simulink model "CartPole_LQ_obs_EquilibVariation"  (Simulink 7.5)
settings: Solver=ode45  StartTime=0.0  StopTime=10.0  MaxStep=1e-2  RelTol=1e-3
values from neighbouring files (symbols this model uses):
  g = 9.81    [Exercises05.m]
  K = lqr(A,B,C'*Q*C,R)    [Exercises05.m]
  L = 1    [Exercises05.m]
  Lobs = - place(A',C',[-20 -20 -25 -25])'    [Exercises05.m]
  m = 0.1    [Exercises05.m]
  M = 1    [Exercises05.m]
  ue = 0    [Exercises05.m]
  X0 = Xe + dX0    [Exercises05.m]
undefined symbols (not defined in the file or in its folder): A, B, C

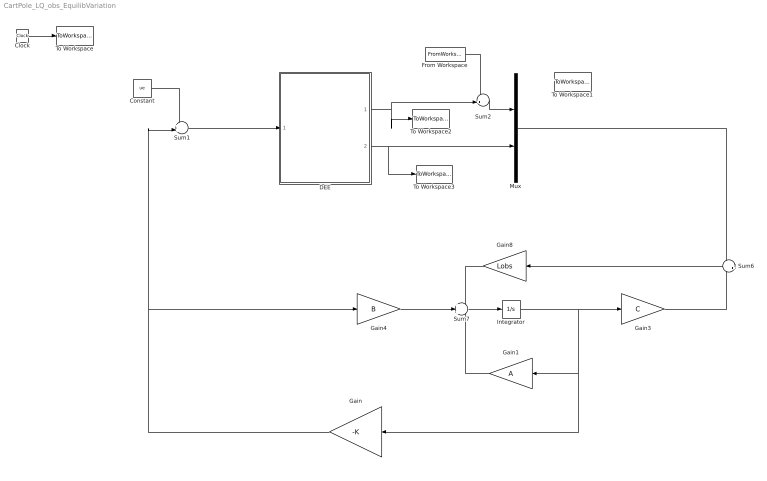
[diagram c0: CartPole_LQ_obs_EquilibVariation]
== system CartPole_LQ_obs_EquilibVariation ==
  Clock : Clock
  Constant : Constant  Value=ue  OutDataType=fixdt(1, 16)  OutScaling=2^0
  DEE : Subsystem
  From Workspace : FromWorkspace  VariableName=[t' Xe_t']  SampleTime=0
  Gain : Gain  Gain=-K  Multiplication=Matrix(K*u)  ParameterDataType=fixdt(1, 16)  ParameterScaling=2^0  OutDataType=fixdt(1, 16)  OutScaling=2^0
  Gain1 : Gain  Gain=A  Multiplication=Matrix(K*u)  ParameterDataType=sfix(16)  ParameterScaling=2^0  OutDataType=sfix(16)  OutScaling=2^0
  Gain3 : Gain  Gain=C  Multiplication=Matrix(K*u)  ParameterDataType=sfix(16)  ParameterScaling=2^0  OutDataType=sfix(16)  OutScaling=2^0
  Gain4 : Gain  Gain=B  Multiplication=Matrix(K*u)  ParameterDataType=sfix(16)  ParameterScaling=2^0  OutDataType=sfix(16)  OutScaling=2^0
  Gain8 : Gain  Gain=Lobs  Multiplication=Matrix(K*u)  ParameterDataType=sfix(16)  ParameterScaling=2^0  OutDataType=sfix(16)  OutScaling=2^0
  Integrator : Integrator  InitialCondition=[0 0 0 0]'
  Mux : Mux  Inputs=2
  Sum1 : Sum  Inputs=++|  OutDataType=fixdt(1, 16)  OutScaling=2^0
  Sum2 : Sum  Inputs=-+|  OutDataType=fixdt(1, 16)  OutScaling=2^0
  Sum6 : Sum  Inputs=-+  OutDataType=sfix(16)  OutScaling=2^0
  Sum7 : Sum  Inputs=+++  OutDataType=sfix(16)  OutScaling=2^0
  To Workspace : ToWorkspace  VariableName=time  SampleTime=-1  SaveFormat=Array
  To Workspace1 : ToWorkspace  VariableName=y  SampleTime=-1  SaveFormat=Array
  To Workspace2 : ToWorkspace  VariableName=y_1  SampleTime=-1  SaveFormat=Array
  To Workspace3 : ToWorkspace  VariableName=y_2  SampleTime=-1  SaveFormat=Array
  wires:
  Clock/1 -> To Workspace/1
  Gain/1 -> Sum1/2, Gain4/1
  Constant/1 -> Sum1/1
  Integrator/1 -> Gain3/1, Gain1/1, Gain/1
  Sum7/1 -> Integrator/1
  Gain3/1 -> Sum6/2
  Sum6/1 -> Gain8/1
  Gain8/1 -> Sum7/1
  Gain1/1 -> Sum7/3
  Gain4/1 -> Sum7/2
  Sum1/1 -> DEE/1(SysInport1)
  DEE/2(Port2) -> Mux/2, To Workspace3/1
  Mux/1 -> Sum6/1
  DEE/1(Port1) -> Sum2/2, To Workspace2/1
  Sum2/1 -> Mux/1
  From Workspace/1 -> Sum2/1

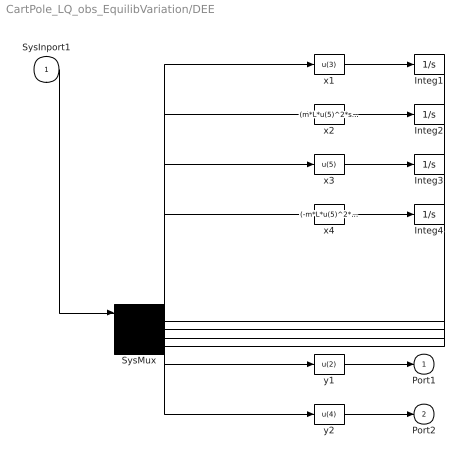
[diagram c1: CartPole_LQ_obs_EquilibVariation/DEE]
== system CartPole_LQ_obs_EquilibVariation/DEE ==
  SysInport1 : Inport
  Integ1 : Integrator  InitialCondition=X0(1)
  Integ2 : Integrator  InitialCondition=X0(2)
  Integ3 : Integrator  InitialCondition=X0(3)
  Integ4 : Integrator  InitialCondition=X0(4)
  SysMux : Mux  Inputs=5
  x1 : Fcn  Expr=u(3)
  x2 : Fcn  Expr=(m*L*u(5)^2*sin(u(4)) - m*g*sin(u(4))*cos(u(4))+ u)/(M+m*sin(u(4))^2)
  x3 : Fcn  Expr=u(5)
  x4 : Fcn  Expr=(-m*L*u(5)^2*sin(u(4))*cos(u(4))+(M+m)*g*sin(u(4))-u*cos(u(4)))/((M+m*sin(u(4))^2)*L)
  y1 : Fcn  Expr=u(2)
  y2 : Fcn  Expr=u(4)
  Port1 : Outport
  Port2 : Outport  Port=2
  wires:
  SysInport1/1 -> SysMux/1
  SysMux/1 -> x1/1, x2/1, x3/1, x4/1, y1/1, y2/1
  x1/1 -> Integ1/1
  Integ1/1 -> SysMux/2
  x2/1 -> Integ2/1
  Integ2/1 -> SysMux/3
  x3/1 -> Integ3/1
  Integ3/1 -> SysMux/4
  x4/1 -> Integ4/1
  Integ4/1 -> SysMux/5
  y1/1 -> Port1/1
  y2/1 -> Port2/1
